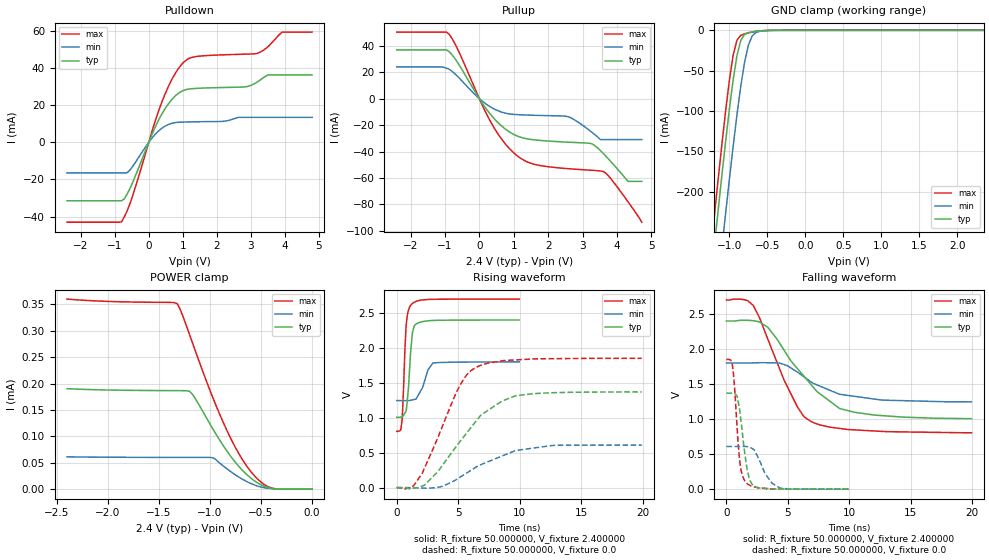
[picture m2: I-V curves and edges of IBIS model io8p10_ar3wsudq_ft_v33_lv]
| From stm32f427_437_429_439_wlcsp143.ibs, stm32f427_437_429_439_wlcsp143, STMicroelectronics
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|   Model io8p10_ar3wsudq_ft_v33_lv
[Model]  io8p10_ar3wsudq_ft_v33_lv
Model_type I/O
Polarity   Non-Inverting
Enable   Active-Low
Vinl =   0.720000V
Vinh =   1.680000V
Vmeas =  1.200000V
Cref =   40.000000pF
Rref =   100.000000M
Vref =   0.0V
C_comp   3.739400pF   3.690400pF   3.817400pF
[Temperature Range]   25.000000   0.125000k   -40.000000
[Pullup Reference]   2.400000V   1.800000V   2.700000V
[Pulldown Reference]   0.0V   0.0V   0.0V
[POWER Clamp Reference]   2.400000V   1.800000V   2.700000V
[GND Clamp Reference]   0.0V   0.0V   0.0V
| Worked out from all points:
|   slope of the pulldown table from 0 to 0.36 V, typ, clamps not added: 25 ohm
|   slope of the pullup table from 0 to 0.36 V, typ, clamps not added: 27.7 ohm
|   GND clamp passes 1 mA (typ) near -0.62 V on its own axis
|   rising waveform, R_fixture 50.000000, V_fixture 2.400000: 20-80 % time 349ps typ, 703ps min, 272ps max; typ from 1.01 V to 2.4 V
|   rising waveform, R_fixture 50.000000, V_fixture 0.0: 20-80 % time 3.81ns typ, 4.15ns min, 2.72ns max; typ from 0 V to 1.37 V
|   falling waveform, R_fixture 50.000000, V_fixture 2.400000: 20-80 % time 4.01ns typ, 3.55ns min, 2.78ns max; typ from 2.4 V to 1.01 V
|   falling waveform, R_fixture 50.000000, V_fixture 0.0: 20-80 % time 600ps typ, 1.08ns min, 462ps max; typ from 1.37 V to 0 V
[Pulldown]
|Voltage   I(typ)   I(min)   I(max)
-2.4V     -31.47mA   -16.45mA   -43.01mA
-800mV    -31.47mA   -16.45mA   -42.85mA
-480mV    -21.98mA   -13.17mA   -29.21mA
80mV      3.63mA     1.966mA    5.014mA
480mV     18.16mA    8.738mA    26.02mA
800mV     25.38mA    10.72mA    37.77mA
1.12V     28.53mA    11.02mA    44.6mA
2.8V      29.84mA    13.49mA    47.53mA
3.2V      32.65mA    13.49mA    48.04mA
3.52V     36.4mA     13.49mA    51.83mA
3.92V     36.4mA     13.49mA    59.44mA
4.8V      36.4mA     13.49mA    59.44mA
[Pullup]
|Voltage   I(typ)   I(min)   I(max)
-2.4V     36.89mA    24.04mA    50.33mA
-960mV    36.89mA    23.05mA    50.33mA
-640mV    27.65mA    17.04mA    37.98mA
320mV     -11.75mA   -6.207mA   -17.08mA
640mV     -20.52mA   -10.1mA    -30.35mA
960mV     -26.47mA   -11.82mA   -40.02mA
1.52V     -30.88mA   -12.51mA   -49.05mA
2.56V     -32.88mA   -13.52mA   -52.9mA
3.28V     -34.25mA   -25.62mA   -54.18mA
3.6V      -41.44mA   -30.97mA   -55.03mA
4.32V     -62.55mA   -30.97mA   -77.98mA
4.72V     -62.55mA   -30.97mA   -93.4mA
[GND_clamp]
|Voltage   I(typ)   I(min)   I(max)
-2.4V     -1.437A    -1.518A    -1.411A
-1.25V    -315.9mA   -407.2mA   -278.2mA
-1.2V     -270.1mA   -361.3mA   -232.1mA
-1.15V    -225mA     -316mA     -186.8mA
-1.1V     -180.9mA   -271.3mA   -142.7mA
-1.05V    -138.2mA   -227.5mA   -100.5mA
-950mV    -61.14mA   -143.6mA   -30.43mA
-900mV    -31.23mA   -104.7mA   -12.14mA
-850mV    -12.49mA   -69.4mA    -6.221mA
-750mV    -2.898mA   -18.35mA   -3.18mA
-600mV    -750.2uA   -1.218mA   -738.3uA
2.35V     0A         0A         0A
[POWER_clamp]
|Voltage   I(typ)   I(min)   I(max)
-2.4V     190.2uA    61.19uA    359.9uA
-1.32V    186.6uA    60.14uA    351.2uA
-1.29V    186.5uA    60.13uA    339.6uA
-1.2V     185.4uA    60.11uA    292.6uA
-1.17V    179.2uA    60.11uA    276.3uA
-960mV    110.2uA    58.62uA    167.5uA
-870mV    82.44uA    43.99uA    126.3uA
-750mV    50.58uA    26.92uA    78.64uA
-630mV    25.94uA    13.41uA    41.02uA
-510mV    9.22uA     4.527uA    14.97uA
-420mV    2.425uA    1.38uA     3.75uA
0V        0A         0A         0A
[Ramp]
| variable   typ   min   max
dV/dt_r  0.82218/3.80846n   0.36559/4.15535n   1.11096/2.71388n
dV/dt_f  0.83394/4.01279n   0.33414/3.67345n   1.13649/2.77628n
R_load = 50.000000
[Rising Waveform]
R_fixture= 50.000000
V_fixture= 2.400000
V_fixture_min= 1.800000
V_fixture_max= 2.700000
|time   V(typ)   V(min)   V(max)
0s        1.006V     1.247V     804.9mV
320.3ps   1.01V      1.247V     821.4mV
440.4ps   1.015V     1.247V     971.8mV
660.7ps   1.066V     1.247V     1.961V
760.8ps   1.095V     1.246V     2.308V
961ps     1.442V     1.246V     2.542V
1.201ns   2.074V     1.254V     2.625V
1.441ns   2.321V     1.262V     2.656V
2.943ns   2.393V     1.785V     2.696V
9.97ns    2.4V       1.8V       2.7V
[Rising Waveform]
R_fixture= 50.000000
V_fixture= 0.0
V_fixture_min= 0.0
V_fixture_max= 0.0
|time   V(typ)   V(min)   V(max)
0s        77.24uV    35.37uV    227.8uV
1.361ns   -8.79mV    -471.8uV   24.32mV
2.082ns   23.76mV    -6.375mV   209.7mV
3.323ns   224.9mV    3.815mV    706.8mV
4.925ns   608.8mV    124.2mV    1.389V
5.646ns   772.3mV    204.4mV    1.604V
6.446ns   950.7mV    293.5mV    1.721V
9.65ns    1.314V     529.7mV    1.828V
12.77ns   1.359V     605.7mV    1.846V
19.94ns   1.37V      609.1mV    1.851V
[Falling Waveform]
R_fixture= 50.000000
V_fixture= 2.400000
V_fixture_min= 1.800000
V_fixture_max= 2.700000
|time   V(typ)   V(min)   V(max)
0s        2.4V       1.8V       2.7V
1.602ns   2.41V      1.8V       2.698V
2.202ns   2.403V     1.802V     2.616V
3.363ns   2.309V     1.805V     2.143V
4.725ns   1.974V     1.776V     1.543V
5.806ns   1.715V     1.667V     1.166V
6.887ns   1.492V     1.531V     966.3mV
9.209ns   1.151V     1.355V     866.9mV
10.41ns   1.098V     1.325V     846mV
19.94ns   1.006V     1.247V     804.9mV
[Falling Waveform]
R_fixture= 50.000000
V_fixture= 0.0
V_fixture_min= 0.0
V_fixture_max= 0.0
|time   V(typ)   V(min)   V(max)
0s        1.37V      609.1mV    1.851V
460.5ps   1.371V     609mV      1.796V
660.7ps   1.367V     608.9mV    1.449V
860.9ps   1.328V     608.8mV    893.3mV
1.181ns   975.9mV    608.6mV    280.9mV
1.622ns   350.9mV    608.1mV    89.08mV
2.242ns   46.35mV    564mV      34.16mV
3.143ns   10.02mV    223.3mV    11.01mV
4.364ns   3.129mV    14.27mV    3.003mV
9.97ns    77.24uV    35.37uV    227.8uV
